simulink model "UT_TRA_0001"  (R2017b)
settings: Solver=FixedStepDiscrete  StartTime=0.0  StopTime=3  FixedStep=0.01  RelTol=1e-3  EnableMultiTasking=on
undefined symbols (not defined in the file): sigbuilder_block

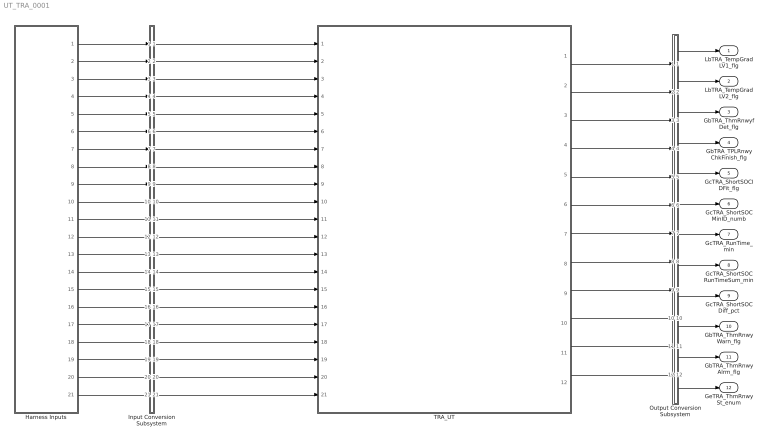
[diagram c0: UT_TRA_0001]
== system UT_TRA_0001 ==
  Harness Inputs : Subsystem  Tag=STV Subsys  LoadFcn=sigbuilder_block('load');  StartFcn=sigbuilder_block('start');  StopFcn=sigbuilder_block('stop');  ClipboardFcn=sigbuilder_block('clipboard');  mask(Sigbuilder block){tuvar=[0:10]}
      mask init:
      | if ~strcmp(get_param(bdroot(gcb),'SimulationStatus'),'stopped'),tuvar = sigbuilder_block('maskInit'); end
  Input Conversion Subsystem : Subsystem  Tag=__SLT_ICS__  Description=Signal spec. and routing
  Output Conversion Subsystem : Subsystem  Tag=__SLT_OCS__  Description=Signal spec. and routing
  TRA_UT : ModelReference  ModelNameDialog=TRA_UT  SimulationMode=Normal  ModelReferenceVersion='M106C107'
  LbTRA_TempGradLV1_flg : Outport  OutDataTypeStr=boolean  PortDimensions=[1]
  LbTRA_TempGradLV2_flg : Outport  Port=2  OutDataTypeStr=boolean  PortDimensions=[1]
  GbTRA_ThmRnwyfDet_flg : Outport  Port=3  OutDataTypeStr=boolean  PortDimensions=[1]
  GbTRA_TPLRnwyChkFinish_flg : Outport  Port=4  OutDataTypeStr=boolean  PortDimensions=[1]
  GcTRA_ShortSOCIDFit_flg : Outport  Port=5  OutDataTypeStr=boolean  PortDimensions=[1]
  GcTRA_ShortSOCMinID_numb : Outport  Port=6  OutDataTypeStr=uint8  PortDimensions=[1]
  GcTRA_RunTime_min : Outport  Port=7  OutDataTypeStr=uint16  PortDimensions=[1]
  GcTRA_ShortSOCRunTimeSum_min : Outport  Port=8  OutDataTypeStr=uint32  PortDimensions=[1]
  GcTRA_ShortSOCDiff_pct : Outport  Port=9  OutDataTypeStr=single  PortDimensions=[1]
  GbTRA_ThmRnwyWarn_flg : Outport  Port=10  OutDataTypeStr=boolean  PortDimensions=[1]
  GbTRA_ThmRnwyAlrm_flg : Outport  Port=11  OutDataTypeStr=boolean  PortDimensions=[1]
  GeTRA_ThmRnwySt_enum : Outport  Port=12  OutDataTypeStr=uint8  PortDimensions=[1]
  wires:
  Harness Inputs/1(GcCDP_MaxCellTemp_C) -> Input Conversion Subsystem/1(Inport_1)
  Harness Inputs/2(GcCDP_MinCellTemp_C) -> Input Conversion Subsystem/2(Inport_2)
  Harness Inputs/3(GcUDS_CellTempNumb_numb) -> Input Conversion Subsystem/3(Inport_3)
  Harness Inputs/4(GcCDP_MaxBusbarTemp_C) -> Input Conversion Subsystem/4(Inport_4)
  Harness Inputs/5(GcCDP_MinBusbarTemp_C) -> Input Conversion Subsystem/5(Inport_5)
  Harness Inputs/6(GcUDS_BusbarTempNumb_numb) -> Input Conversion Subsystem/6(Inport_6)
  Harness Inputs/7(GeMSM_BMUState_enum) -> Input Conversion Subsystem/7(Inport_7)
  Harness Inputs/8(GbCDP_SumCellVoltVld_flg) -> Input Conversion Subsystem/8(Inport_8)
  Harness Inputs/9(GcRTC_SleepTime_min) -> Input Conversion Subsystem/9(Inport_9)
  Harness Inputs/10(GbNDP_ReadShortSOCIDFitVld_flg) -> Input Conversion Subsystem/10(Inport_10)
  Harness Inputs/11(GbISP_ReadShortSOCIDFit_flg) -> Input Conversion Subsystem/11(Inport_11)
  Harness Inputs/12(GbNDP_ReadShortSOCMinIDVld_flg) -> Input Conversion Subsystem/12(Inport_12)
  Harness Inputs/13(GcISP_ShortSOCMinID_numb) -> Input Conversion Subsystem/13(Inport_13)
  Harness Inputs/14(GbNDP_ReadShortSOCDiffVld_flg) -> Input Conversion Subsystem/14(Inport_14)
  Harness Inputs/15(GcISP_ShortSOCDiff_pct) -> Input Conversion Subsystem/15(Inport_15)
  Harness Inputs/16(GbNDP_ReadShortSOCRunTiSumVld_flg) -> Input Conversion Subsystem/16(Inport_16)
  Harness Inputs/17(GcISP_ShortSOCRunTiSum_min) -> Input Conversion Subsystem/17(Inport_17)
  Harness Inputs/18(GeUDS_CapSel_enum) -> Input Conversion Subsystem/18(Inport_18)
  Harness Inputs/19(GcISP_LastShortSOCRunTiVld_flg) -> Input Conversion Subsystem/19(Inport_19)
  Harness Inputs/20(GcISP_LastShortSOCRunTi_min) -> Input Conversion Subsystem/20(Inport_20)
  Harness Inputs/21(GcCDP_AvgCellVolt_mV) -> Input Conversion Subsystem/21(Inport_21)
  Output Conversion Subsystem/1(Outport_1) -> LbTRA_TempGradLV1_flg/1
  Output Conversion Subsystem/2(Outport_2) -> LbTRA_TempGradLV2_flg/1
  Output Conversion Subsystem/3(Outport_3) -> GbTRA_ThmRnwyfDet_flg/1
  Output Conversion Subsystem/4(Outport_4) -> GbTRA_TPLRnwyChkFinish_flg/1
  Output Conversion Subsystem/5(Outport_5) -> GcTRA_ShortSOCIDFit_flg/1
  Output Conversion Subsystem/6(Outport_6) -> GcTRA_ShortSOCMinID_numb/1
  Output Conversion Subsystem/7(Outport_7) -> GcTRA_RunTime_min/1
  Output Conversion Subsystem/8(Outport_8) -> GcTRA_ShortSOCRunTimeSum_min/1
  Output Conversion Subsystem/9(Outport_9) -> GcTRA_ShortSOCDiff_pct/1
  Output Conversion Subsystem/10(Outport_10) -> GbTRA_ThmRnwyWarn_flg/1
  Output Conversion Subsystem/11(Outport_11) -> GbTRA_ThmRnwyAlrm_flg/1
  Output Conversion Subsystem/12(Outport_12) -> GeTRA_ThmRnwySt_enum/1
  Input Conversion Subsystem/1(Outport_1) -> TRA_UT/1
  Input Conversion Subsystem/2(Outport_2) -> TRA_UT/2
  Input Conversion Subsystem/3(Outport_3) -> TRA_UT/3
  Input Conversion Subsystem/4(Outport_4) -> TRA_UT/4
  Input Conversion Subsystem/5(Outport_5) -> TRA_UT/5
  Input Conversion Subsystem/6(Outport_6) -> TRA_UT/6
  Input Conversion Subsystem/7(Outport_7) -> TRA_UT/7
  Input Conversion Subsystem/8(Outport_8) -> TRA_UT/8
  Input Conversion Subsystem/9(Outport_9) -> TRA_UT/9
  Input Conversion Subsystem/10(Outport_10) -> TRA_UT/10
  Input Conversion Subsystem/11(Outport_11) -> TRA_UT/11
  Input Conversion Subsystem/12(Outport_12) -> TRA_UT/12
  Input Conversion Subsystem/13(Outport_13) -> TRA_UT/13
  Input Conversion Subsystem/14(Outport_14) -> TRA_UT/14
  Input Conversion Subsystem/15(Outport_15) -> TRA_UT/15
  Input Conversion Subsystem/16(Outport_16) -> TRA_UT/16
  Input Conversion Subsystem/17(Outport_17) -> TRA_UT/17
  Input Conversion Subsystem/18(Outport_18) -> TRA_UT/18
  Input Conversion Subsystem/19(Outport_19) -> TRA_UT/19
  Input Conversion Subsystem/20(Outport_20) -> TRA_UT/20
  Input Conversion Subsystem/21(Outport_21) -> TRA_UT/21
  TRA_UT/1 -> Output Conversion Subsystem/1(Inport_1)
  TRA_UT/2 -> Output Conversion Subsystem/2(Inport_2)
  TRA_UT/3 -> Output Conversion Subsystem/3(Inport_3)
  TRA_UT/4 -> Output Conversion Subsystem/4(Inport_4)
  TRA_UT/5 -> Output Conversion Subsystem/5(Inport_5)
  TRA_UT/6 -> Output Conversion Subsystem/6(Inport_6)
  TRA_UT/7 -> Output Conversion Subsystem/7(Inport_7)
  TRA_UT/8 -> Output Conversion Subsystem/8(Inport_8)
  TRA_UT/9 -> Output Conversion Subsystem/9(Inport_9)
  TRA_UT/10 -> Output Conversion Subsystem/10(Inport_10)
  TRA_UT/11 -> Output Conversion Subsystem/11(Inport_11)
  TRA_UT/12 -> Output Conversion Subsystem/12(Inport_12)

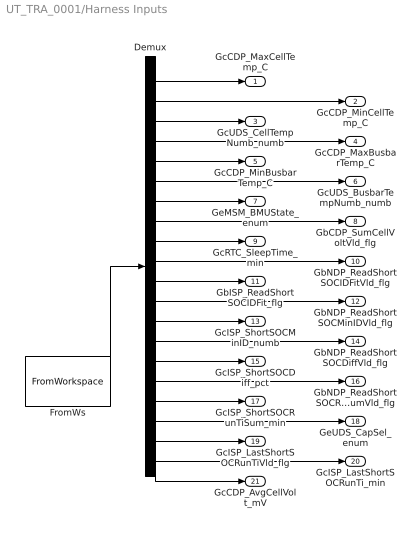
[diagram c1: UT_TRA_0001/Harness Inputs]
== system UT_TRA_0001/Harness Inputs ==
  Demux : Demux  Tag=STV Demux  Outputs=21
  FromWs : FromWorkspace  Tag=STV FromWs  VariableName=tuvar  SampleTime=0
  GcCDP_MaxCellTemp_C : Outport  Tag=STV Outport
  GcCDP_MinCellTemp_C : Outport  Tag=STV Outport  Port=2
  GcUDS_CellTempNumb_numb : Outport  Tag=STV Outport  Port=3
  GcCDP_MaxBusbarTemp_C : Outport  Tag=STV Outport  Port=4
  GcCDP_MinBusbarTemp_C : Outport  Tag=STV Outport  Port=5
  GcUDS_BusbarTempNumb_numb : Outport  Tag=STV Outport  Port=6
  GeMSM_BMUState_enum : Outport  Tag=STV Outport  Port=7
  GbCDP_SumCellVoltVld_flg : Outport  Tag=STV Outport  Port=8
  GcRTC_SleepTime_min : Outport  Tag=STV Outport  Port=9
  GbNDP_ReadShortSOCIDFitVld_flg : Outport  Tag=STV Outport  Port=10
  GbISP_ReadShortSOCIDFit_flg : Outport  Tag=STV Outport  Port=11
  GbNDP_ReadShortSOCMinIDVld_flg : Outport  Tag=STV Outport  Port=12
  GcISP_ShortSOCMinID_numb : Outport  Tag=STV Outport  Port=13
  GbNDP_ReadShortSOCDiffVld_flg : Outport  Tag=STV Outport  Port=14
  GcISP_ShortSOCDiff_pct : Outport  Tag=STV Outport  Port=15
  GbNDP_ReadShortSOCRunTiSumVld_flg : Outport  Tag=STV Outport  Port=16
  GcISP_ShortSOCRunTiSum_min : Outport  Tag=STV Outport  Port=17
  GeUDS_CapSel_enum : Outport  Tag=STV Outport  Port=18
  GcISP_LastShortSOCRunTiVld_flg : Outport  Tag=STV Outport  Port=19
  GcISP_LastShortSOCRunTi_min : Outport  Tag=STV Outport  Port=20
  GcCDP_AvgCellVolt_mV : Outport  Tag=STV Outport  Port=21
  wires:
  FromWs/1 -> Demux/1
  Demux/1 -> GcCDP_MaxCellTemp_C/1
  Demux/2 -> GcCDP_MinCellTemp_C/1
  Demux/3 -> GcUDS_CellTempNumb_numb/1
  Demux/4 -> GcCDP_MaxBusbarTemp_C/1
  Demux/5 -> GcCDP_MinBusbarTemp_C/1
  Demux/6 -> GcUDS_BusbarTempNumb_numb/1
  Demux/7 -> GeMSM_BMUState_enum/1
  Demux/8 -> GbCDP_SumCellVoltVld_flg/1
  Demux/9 -> GcRTC_SleepTime_min/1
  Demux/10 -> GbNDP_ReadShortSOCIDFitVld_flg/1
  Demux/11 -> GbISP_ReadShortSOCIDFit_flg/1
  Demux/12 -> GbNDP_ReadShortSOCMinIDVld_flg/1
  Demux/13 -> GcISP_ShortSOCMinID_numb/1
  Demux/14 -> GbNDP_ReadShortSOCDiffVld_flg/1
  Demux/15 -> GcISP_ShortSOCDiff_pct/1
  Demux/16 -> GbNDP_ReadShortSOCRunTiSumVld_flg/1
  Demux/17 -> GcISP_ShortSOCRunTiSum_min/1
  Demux/18 -> GeUDS_CapSel_enum/1
  Demux/19 -> GcISP_LastShortSOCRunTiVld_flg/1
  Demux/20 -> GcISP_LastShortSOCRunTi_min/1
  Demux/21 -> GcCDP_AvgCellVolt_mV/1

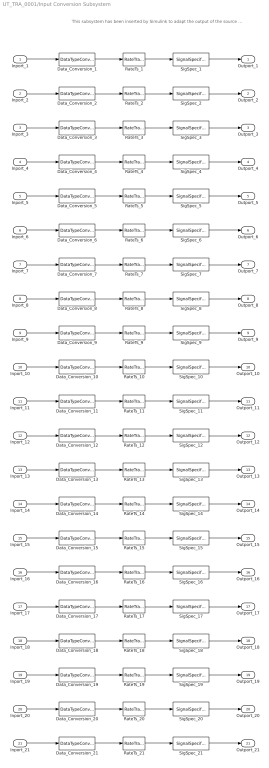
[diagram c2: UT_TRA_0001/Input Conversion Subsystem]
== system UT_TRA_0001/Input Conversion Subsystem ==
  note: This subsystem has been inserted by Simulink to adapt the output of the source blocks to the interface required by the harnessed component. Modifying the contents of this subsystem may result in compilation and simulation failure.
  Inport_1 : Inport
  Inport_2 : Inport  Port=2
  Inport_3 : Inport  Port=3
  Inport_4 : Inport  Port=4
  Inport_5 : Inport  Port=5
  Inport_6 : Inport  Port=6
  Inport_7 : Inport  Port=7
  Inport_8 : Inport  Port=8
  Inport_9 : Inport  Port=9
  Inport_10 : Inport  Port=10
  Inport_11 : Inport  Port=11
  Inport_12 : Inport  Port=12
  Inport_13 : Inport  Port=13
  Inport_14 : Inport  Port=14
  Inport_15 : Inport  Port=15
  Inport_16 : Inport  Port=16
  Inport_17 : Inport  Port=17
  Inport_18 : Inport  Port=18
  Inport_19 : Inport  Port=19
  Inport_20 : Inport  Port=20
  Inport_21 : Inport  Port=21
  Data_Conversion_{1..2,4..5,15} (5 alike) : DataTypeConversion  OutDataTypeStr=single
  Data_Conversion_{8,10..12,14,16,19} (7 alike) : DataTypeConversion  OutDataTypeStr=boolean
  Data_Conversion_{3,6..7,13,18} (5 alike) : DataTypeConversion  OutDataTypeStr=uint8
  Data_Conversion_17 : DataTypeConversion  OutDataTypeStr=uint32
  Data_Conversion_20 : DataTypeConversion  OutDataTypeStr=uint16
  Data_Conversion_21 : DataTypeConversion  OutDataTypeStr=uint16
  Data_Conversion_9 : DataTypeConversion  OutDataTypeStr=uint32
  RateTs_{1..21} (21 alike) : RateTransition  OutPortSampleTime=0.01
  SigSpec_{1..2,4..5} (4 alike) : SignalSpecification  OutDataTypeStr=single  Unit=C  Dimensions=[1]  SampleTime=0.01
  SigSpec_{8,10..12,14,16,19} (7 alike) : SignalSpecification  OutDataTypeStr=boolean  Unit=flag  Dimensions=[1]  SampleTime=0.01
  SigSpec_13 : SignalSpecification  OutDataTypeStr=uint8  Unit=numb  Dimensions=[1]  SampleTime=0.01
  SigSpec_15 : SignalSpecification  OutDataTypeStr=single  Unit=pct  Dimensions=[1]  SampleTime=0.01
  SigSpec_17 : SignalSpecification  OutDataTypeStr=uint32  Unit=min  Dimensions=[1]  SampleTime=0.01
  SigSpec_18 : SignalSpecification  OutDataTypeStr=uint8  Unit=enum  Dimensions=[1]  SampleTime=0.01
  SigSpec_20 : SignalSpecification  OutDataTypeStr=uint16  Unit=min  Dimensions=[1]  SampleTime=0.01
  SigSpec_21 : SignalSpecification  OutDataTypeStr=uint16  Unit=mV  Dimensions=[1]  SampleTime=0.01
  SigSpec_3 : SignalSpecification  OutDataTypeStr=uint8  Unit=numb  Dimensions=[1]  SampleTime=0.01
  SigSpec_6 : SignalSpecification  OutDataTypeStr=uint8  Unit=numb  Dimensions=[1]  SampleTime=0.01
  SigSpec_7 : SignalSpecification  OutDataTypeStr=uint8  Unit=enum  Dimensions=[1]  SampleTime=0.01
  SigSpec_9 : SignalSpecification  OutDataTypeStr=uint32  Unit=min  Dimensions=[1]  SampleTime=0.01
  Outport_1 : Outport
  Outport_2 : Outport  Port=2
  Outport_3 : Outport  Port=3
  Outport_4 : Outport  Port=4
  Outport_5 : Outport  Port=5
  Outport_6 : Outport  Port=6
  Outport_7 : Outport  Port=7
  Outport_8 : Outport  Port=8
  Outport_9 : Outport  Port=9
  Outport_10 : Outport  Port=10
  Outport_11 : Outport  Port=11
  Outport_12 : Outport  Port=12
  Outport_13 : Outport  Port=13
  Outport_14 : Outport  Port=14
  Outport_15 : Outport  Port=15
  Outport_16 : Outport  Port=16
  Outport_17 : Outport  Port=17
  Outport_18 : Outport  Port=18
  Outport_19 : Outport  Port=19
  Outport_20 : Outport  Port=20
  Outport_21 : Outport  Port=21
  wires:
  SigSpec_1/1 -> Outport_1/1
  RateTs_1/1 -> SigSpec_1/1
  Data_Conversion_1/1 -> RateTs_1/1
  Inport_1/1 -> Data_Conversion_1/1
  SigSpec_2/1 -> Outport_2/1
  RateTs_2/1 -> SigSpec_2/1
  Data_Conversion_2/1 -> RateTs_2/1
  Inport_2/1 -> Data_Conversion_2/1
  SigSpec_3/1 -> Outport_3/1
  RateTs_3/1 -> SigSpec_3/1
  Data_Conversion_3/1 -> RateTs_3/1
  Inport_3/1 -> Data_Conversion_3/1
  SigSpec_4/1 -> Outport_4/1
  RateTs_4/1 -> SigSpec_4/1
  Data_Conversion_4/1 -> RateTs_4/1
  Inport_4/1 -> Data_Conversion_4/1
  SigSpec_5/1 -> Outport_5/1
  RateTs_5/1 -> SigSpec_5/1
  Data_Conversion_5/1 -> RateTs_5/1
  Inport_5/1 -> Data_Conversion_5/1
  SigSpec_6/1 -> Outport_6/1
  RateTs_6/1 -> SigSpec_6/1
  Data_Conversion_6/1 -> RateTs_6/1
  Inport_6/1 -> Data_Conversion_6/1
  SigSpec_7/1 -> Outport_7/1
  RateTs_7/1 -> SigSpec_7/1
  Data_Conversion_7/1 -> RateTs_7/1
  Inport_7/1 -> Data_Conversion_7/1
  SigSpec_8/1 -> Outport_8/1
  RateTs_8/1 -> SigSpec_8/1
  Data_Conversion_8/1 -> RateTs_8/1
  Inport_8/1 -> Data_Conversion_8/1
  SigSpec_9/1 -> Outport_9/1
  RateTs_9/1 -> SigSpec_9/1
  Data_Conversion_9/1 -> RateTs_9/1
  Inport_9/1 -> Data_Conversion_9/1
  SigSpec_10/1 -> Outport_10/1
  RateTs_10/1 -> SigSpec_10/1
  Data_Conversion_10/1 -> RateTs_10/1
  Inport_10/1 -> Data_Conversion_10/1
  SigSpec_11/1 -> Outport_11/1
  RateTs_11/1 -> SigSpec_11/1
  Data_Conversion_11/1 -> RateTs_11/1
  Inport_11/1 -> Data_Conversion_11/1
  SigSpec_12/1 -> Outport_12/1
  RateTs_12/1 -> SigSpec_12/1
  Data_Conversion_12/1 -> RateTs_12/1
  Inport_12/1 -> Data_Conversion_12/1
  SigSpec_13/1 -> Outport_13/1
  RateTs_13/1 -> SigSpec_13/1
  Data_Conversion_13/1 -> RateTs_13/1
  Inport_13/1 -> Data_Conversion_13/1
  SigSpec_14/1 -> Outport_14/1
  RateTs_14/1 -> SigSpec_14/1
  Data_Conversion_14/1 -> RateTs_14/1
  Inport_14/1 -> Data_Conversion_14/1
  SigSpec_15/1 -> Outport_15/1
  RateTs_15/1 -> SigSpec_15/1
  Data_Conversion_15/1 -> RateTs_15/1
  Inport_15/1 -> Data_Conversion_15/1
  SigSpec_16/1 -> Outport_16/1
  RateTs_16/1 -> SigSpec_16/1
  Data_Conversion_16/1 -> RateTs_16/1
  Inport_16/1 -> Data_Conversion_16/1
  SigSpec_17/1 -> Outport_17/1
  RateTs_17/1 -> SigSpec_17/1
  Data_Conversion_17/1 -> RateTs_17/1
  Inport_17/1 -> Data_Conversion_17/1
  SigSpec_18/1 -> Outport_18/1
  RateTs_18/1 -> SigSpec_18/1
  Data_Conversion_18/1 -> RateTs_18/1
  Inport_18/1 -> Data_Conversion_18/1
  SigSpec_19/1 -> Outport_19/1
  RateTs_19/1 -> SigSpec_19/1
  Data_Conversion_19/1 -> RateTs_19/1
  Inport_19/1 -> Data_Conversion_19/1
  SigSpec_20/1 -> Outport_20/1
  RateTs_20/1 -> SigSpec_20/1
  Data_Conversion_20/1 -> RateTs_20/1
  Inport_20/1 -> Data_Conversion_20/1
  SigSpec_21/1 -> Outport_21/1
  RateTs_21/1 -> SigSpec_21/1
  Data_Conversion_21/1 -> RateTs_21/1
  Inport_21/1 -> Data_Conversion_21/1

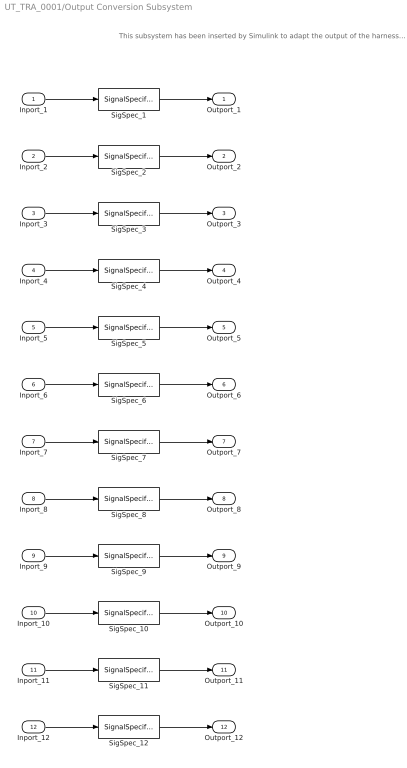
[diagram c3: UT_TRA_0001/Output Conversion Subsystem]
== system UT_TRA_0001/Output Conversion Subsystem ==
  note: This subsystem has been inserted by Simulink to adapt the output of the harnessed component to the interface required by the sink blocks. Modifying the contents of this subsystem may result in compilation and simulation failure.
  Inport_1 : Inport
  Inport_2 : Inport  Port=2
  Inport_3 : Inport  Port=3
  Inport_4 : Inport  Port=4
  Inport_5 : Inport  Port=5
  Inport_6 : Inport  Port=6
  Inport_7 : Inport  Port=7
  Inport_8 : Inport  Port=8
  Inport_9 : Inport  Port=9
  Inport_10 : Inport  Port=10
  Inport_11 : Inport  Port=11
  Inport_12 : Inport  Port=12
  SigSpec_{1..5,10..11} (7 alike) : SignalSpecification  OutDataTypeStr=boolean  Unit=flag  Dimensions=[1]  SampleTime=0.01
  SigSpec_12 : SignalSpecification  OutDataTypeStr=uint8  Unit=enum  Dimensions=[1]  SampleTime=0.01
  SigSpec_6 : SignalSpecification  OutDataTypeStr=uint8  Unit=numb  Dimensions=[1]  SampleTime=0.01
  SigSpec_7 : SignalSpecification  OutDataTypeStr=uint16  Unit=min  Dimensions=[1]  SampleTime=0.01
  SigSpec_8 : SignalSpecification  OutDataTypeStr=uint32  Unit=min  Dimensions=[1]  SampleTime=0.01
  SigSpec_9 : SignalSpecification  OutDataTypeStr=single  Unit=pct  Dimensions=[1]  SampleTime=0.01
  Outport_1 : Outport
  Outport_2 : Outport  Port=2
  Outport_3 : Outport  Port=3
  Outport_4 : Outport  Port=4
  Outport_5 : Outport  Port=5
  Outport_6 : Outport  Port=6
  Outport_7 : Outport  Port=7
  Outport_8 : Outport  Port=8
  Outport_9 : Outport  Port=9
  Outport_10 : Outport  Port=10
  Outport_11 : Outport  Port=11
  Outport_12 : Outport  Port=12
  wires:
  Inport_1/1 -> SigSpec_1/1
  SigSpec_1/1 -> Outport_1/1
  Inport_2/1 -> SigSpec_2/1
  SigSpec_2/1 -> Outport_2/1
  Inport_3/1 -> SigSpec_3/1
  SigSpec_3/1 -> Outport_3/1
  Inport_4/1 -> SigSpec_4/1
  SigSpec_4/1 -> Outport_4/1
  Inport_5/1 -> SigSpec_5/1
  SigSpec_5/1 -> Outport_5/1
  Inport_6/1 -> SigSpec_6/1
  SigSpec_6/1 -> Outport_6/1
  Inport_7/1 -> SigSpec_7/1
  SigSpec_7/1 -> Outport_7/1
  Inport_8/1 -> SigSpec_8/1
  SigSpec_8/1 -> Outport_8/1
  Inport_9/1 -> SigSpec_9/1
  SigSpec_9/1 -> Outport_9/1
  Inport_10/1 -> SigSpec_10/1
  SigSpec_10/1 -> Outport_10/1
  Inport_11/1 -> SigSpec_11/1
  SigSpec_11/1 -> Outport_11/1
  Inport_12/1 -> SigSpec_12/1
  SigSpec_12/1 -> Outport_12/1
